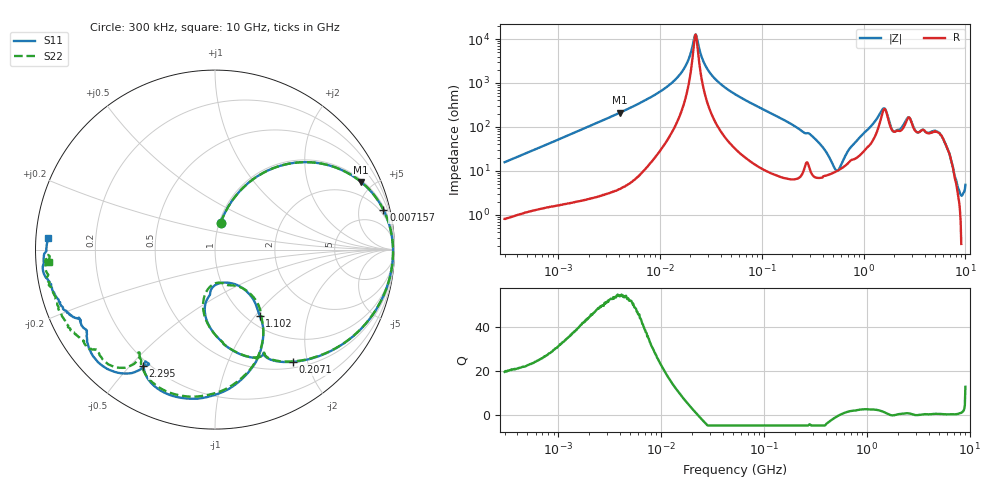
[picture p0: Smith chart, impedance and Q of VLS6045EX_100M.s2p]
! S-Parameter Data Generated by TDK Corporation
! Copyright(C) 2019 TDK Corporation.
! All Rights Reserved.
! TDK P/N: VLS6045EX-100M (Inductor)
! Property: L=10uH at 100kHz
! Size(LxWxT): 6x6x4.5mm
! Model Type: s2p (Touchstone File Format Version 1.0)
! Frequency: DC=Yes Start=0.3MHz Stop=10000MHz 802points Log-sweep
! Model Generated on May 10, 2019
! Port Assignments:
!  1 ---@@@--- 2
! Applicable Conditions:
!  Temperature = 25 degC
!  DC Bias Current = 0 A
!  Small Signal Operation
! Terms and conditions regarding TDK Simulation Models
! (1)This simulation model is being provided solely for informational purposes. Please refer to the specifications of the products in terms of detailed characteristics of such products.
! (2)In no event shall TDK Corporation of any of its subsidiaries be liable for any loss or damage arising, directly or indirectly,
!  From any information contained in this simulation model, including, but not limited to loss or damages arising from any inaccuracies, omissions or errors in connection with such information.
! (3)Any and all copyrights on this simulation model are owned by TDK Corporation.
!  Duplication or redistribution of this simulation model without prior written permission from TDK Corporation is prohibited.
! (4)This simulation model is subject to any modification or change without any prior notice.
! (5)Neither TDK Corporation nor any of its subsidiaries shall make any warranty, express or implied,
!  Including but not limited to the correctness, implied warranties of merchantability and fitness for a particular purpose with respect to this simulation models.
! (6)The use of this simulation model shall be deemed to have consented to the terms and conditions hereof.
# Hz S MA R 50
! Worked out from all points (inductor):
!   801 points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, 300 kHz to 10 GHz, reference 50 ohm
!   read as one part in series: L = 8.27 uH near 318.3 kHz
!   highest Q = 54.2 at 4.054 MHz (marker M1), where L = 8.26 uH
!   self-resonance near 22.21 MHz
!   S11 on the Smith chart (normalised r, x): 300 kHz: 1.02, +0.31; 7.157 MHz: 1.33, +8.37; 207.1 MHz: 0.59, -1.76; 1.102 GHz: 1.15, -1.06; 2.295 GHz: 0.18, -0.55; 10 GHz: 0.04, +0.03
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300000  0.153 78.2  0.9802 -8.9  0.9805 -8.9  0.1527 78.0
1713600  0.6483 48.1  0.7459 -40.6  0.7461 -40.6  0.6482 48.1
4053600  0.8966 24.9  0.4267 -64.0  0.4267 -64.0  0.8966 24.9
7156657  0.9642 13.3  0.2404 -75.2  0.2404 -75.2  0.9643 13.3
9671944  0.9796 8.6  0.1636 -79.0  0.1636 -79.0  0.9797 8.6
1.649435e7  0.991 1.7  0.05535 -80.5  0.05537 -80.5  0.991 1.7
2.252362e7  0.9921 -2.0  0.007806 0.9  0.007805 0.9  0.9922 -1.9
3.075078e7  0.9901 -5.8  0.05613 75.8  0.05614 75.8  0.9902 -5.8
5.477226e7  0.9748 -14.7  0.1737 72.1  0.1737 72.1  0.9749 -14.6
2.070906e8  0.7614 -55.2  0.6089 32.0  0.6088 32.0  0.7618 -54.8
3.126428e8  0.6324 -71.6  0.7142 12.8  0.7142 12.8  0.6325 -71.4
5.046115e8  0.4126 -95.5  0.8255 -17.2  0.8254 -17.2  0.4072 -96.3
7.400828e8  0.2449 -96.3  0.7901 -49.4  0.7901 -49.4  0.1851 -85.3
8.643532e8  0.1982 -68.5  0.768 -64.6  0.7679 -64.6  0.2263 -62.3
1.10164e9  0.4459 -55.9  0.5868 -96.7  0.5867 -96.7  0.4716 -56.2
1.591286e9  0.8443 -100.6  0.1305 -105.9  0.1308 -105.7  0.8341 -101.9
1.767019e9  0.8306 -114.3  0.168 -76.0  0.1687 -76.1  0.8183 -115.1
2.294622e9  0.7632 -121.6  0.2123 -113.9  0.2127 -114.2  0.7111 -126.2
2.798208e9  0.9003 -133.7  0.08992 -119.0  0.0899 -119.4  0.863 -130.9
3.387826e9  0.8557 -146.5  0.1224 -114.6  0.1219 -114.9  0.8612 -139.6
5.849356e9  0.9165 -161.6  0.04791 -138.8  0.0479 -138.3  0.9322 -158.1
1e10  0.931 176.2  0.04436 -153.9  0.04451 -154.1  0.9275 -175.8
